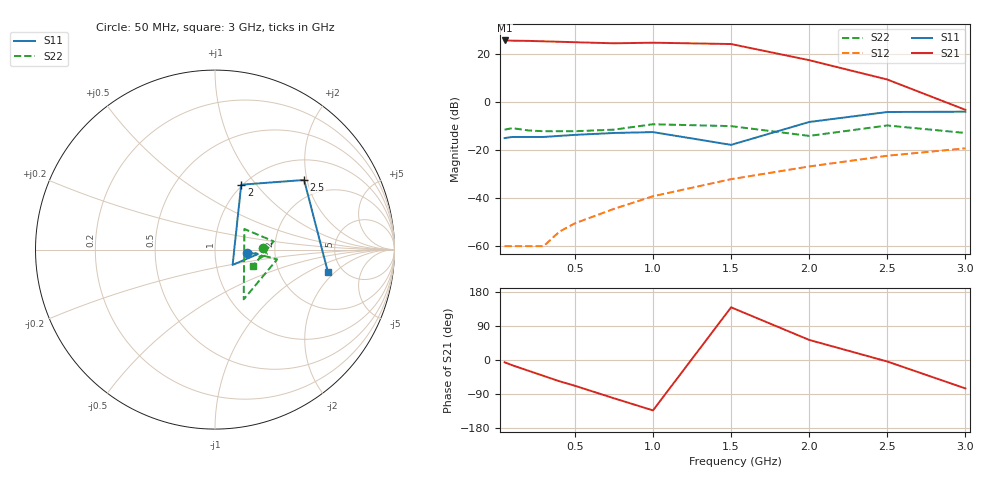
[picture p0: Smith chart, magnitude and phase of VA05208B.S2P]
!  IVA-05208  S PARAMETERS
!  S PARAMETERS (VGC=3.4V, Id=32.6 mA)  LAST UPDATED 08-11-93
# ghz s ma r 50
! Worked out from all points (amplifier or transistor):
!   12 points, 50 MHz to 3 GHz, reference 50 ohm
!   highest |S21| = 25.8 dB at 50 MHz (marker M1)
!   |S21| within 3 dB of that: start of sweep to 1.612 GHz
!   unconditionally stable (mu >= 1): start of sweep to end of sweep
!   at 200 MHz: K = 23.41, MAG = 26.1 dB, |S12| = -60.0 dB
!   at 750 MHz: K = 4.29, MAG = 25.3 dB, |S12| = -44.4 dB
!   at 3 GHz: K = 3.53, MAG = -0.4 dB, |S12| = -19.2 dB
!   S11 on the Smith chart (normalised r, x): 50 MHz: 1.43, -0.06; 2 GHz: 0.99, +0.84; 2.5 GHz: 1.49, +1.92; 3 GHz: 3.86, -1.60
0.05  0.18 -6.0  19.6 -6.0  0.001 48.0  0.27 2.0
0.1  0.19 -6.0  19.4 -14.0  0.001 66.0  0.29 -5.0
0.2  0.19 -5.0  19.2 -28.0  0.001 96.0  0.26 -10.0
0.3  0.19 -3.0  18.8 -42.0  0.001 114.0  0.25 -9.0
0.4  0.2 -3.0  18.4 -56.0  0.002 111.0  0.25 -9.0
0.5  0.21 -6.0  18 -68.0  0.003 117.0  0.25 -9.0
0.75  0.23 -5.0  17.1 -101.0  0.006 135.0  0.27 -7.0
1  0.24 -6.0  17.6 -133.0  0.011 138.0  0.35 -9.0
1.5  0.13 -41.0  16.5 139.0  0.025 121.0  0.32 -60.0
2  0.39 68.0  7.6 53.0  0.046 110.0  0.2 35.0
2.5  0.63 38.0  3 -4.0  0.077 95.0  0.33 8.0
3  0.64 -11.0  0.7 -75.0  0.11 62.0  0.23 -23.0
